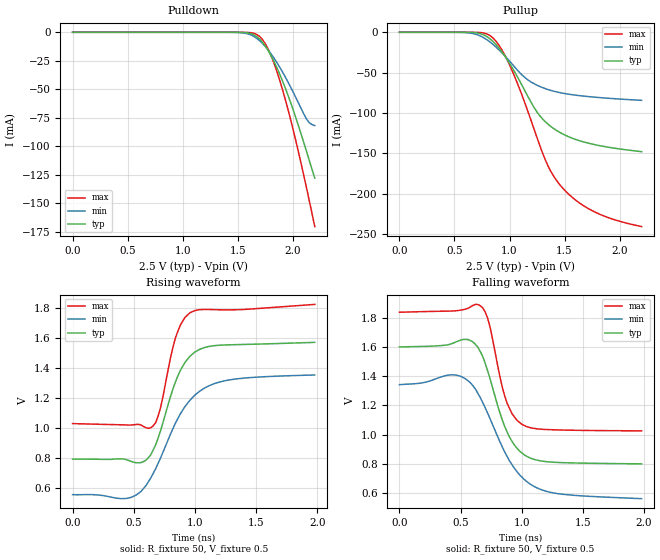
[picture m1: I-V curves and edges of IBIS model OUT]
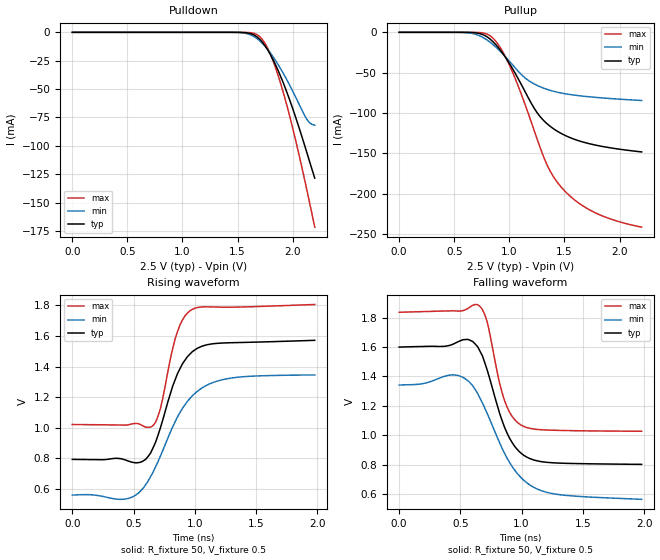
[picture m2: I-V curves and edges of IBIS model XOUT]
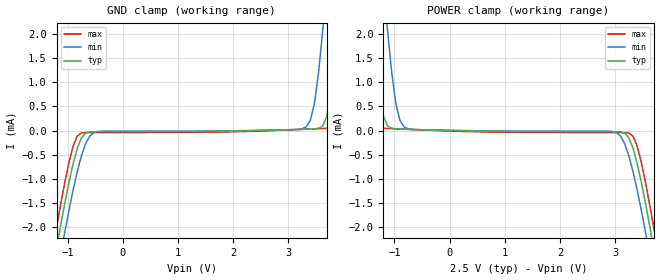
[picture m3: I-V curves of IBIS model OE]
|   IBIS File sg3225ean_25v.ibs
[IBIS Ver]   3.2
[File name]   sg3225ean_25v.ibs
[File Rev]   1.0
[Date]   May 1, 2013
[Source]
[Disclaimer]
Seiko Epson Corporation makes no warranty with respect to the information
contained herein.
[Copyright]
Copyright(C) 2013, Seiko Epson Corporation. All rights reserved.
|   Component SG3225EAN 2.5V
[Component]   sg3225ean_25v
[Manufacturer]   Seiko Epson Corporation
[Package]
R_pkg   0.048   NA   NA
L_pkg   0.48n   NA   NA
C_pkg   0.21p   NA   NA
[Pin] signal_name   model_name   R_pin   L_pin   C_pin
1   OE   OE
2   GND   GND
3   GND   GND
4   OUT   OUT   0.048   0.48n   0.21p
5   XOUT   XOUT   0.048   0.48n   0.21p
6   VCC   POWER
[Diff Pin] inv_pin vdiff   tdelay_typ
4   5   0   0
| Models and submodels in the file (3): OUT (Output_ECL), XOUT (Output_ECL), OE (Input)
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[Model]   OUT
Model_type Output_ECL
Enable Active-High
Polarity Non-Inverting
Vref=0.5
Vmeas=1.17
Rref=50
Cref=0
C_comp   0.121p   0.121p   0.121p
[Temperature Range] 25   105   -40
[Voltage Range]   2.5   2.25   2.75
[Pullup Reference]  2.5   2.25   2.75
[Pulldown Reference]2.5   2.25   2.75
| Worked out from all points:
|   falling waveform, R_fixture 50, V_fixture 0.5: 20-80 % time 196ps typ, 291ps min, 139ps max; typ from 1.6 V to 0.802 V
|   rising waveform, R_fixture 50, V_fixture 0.5: 20-80 % time 197ps typ, 299ps min, 137ps max; typ from 0.794 V to 1.57 V
[Pullup]
0V        611pA      1.028nA    671.3pA
625mV     -80.21uA   -627.6uA   -4.517uA
825mV     -8.344mA   -12.23mA   -4.283mA
900mV     -18.9mA    -21.18mA   -15.25mA
1V        -38.41mA   -35.67mA   -40.23mA
1.125V    -68.68mA   -54.32mA   -82.25mA
1.25V     -98.86mA   -65.59mA   -130.6mA
1.35V     -113.9mA   -70.95mA   -165.7mA
1.45V     -123.5mA   -74.53mA   -187.7mA
1.575V    -131.5mA   -77.43mA   -205.1mA
1.75V     -138.5mA   -80.07mA   -220.9mA
2.2V      -147.9mA   -84.31mA   -240.7mA
[Pulldown]
0V        611.1pA    1.029nA    671.4pA
1.5V      -32.97uA   -162.8uA   -2.785uA
1.625V    -1.356mA   -2.54mA    -453.5uA
1.7V      -6.054mA   -7.439mA   -3.728mA
1.75V     -12.01mA   -12.41mA   -9.925mA
1.8V      -20.03mA   -18.54mA   -19.8mA
1.85V     -29.76mA   -25.66mA   -32.69mA
1.9V      -40.95mA   -33.63mA   -47.96mA
2V        -66.91mA   -51.72mA   -83.97mA
2.125V    -104.4mA   -76.02mA   -136.4mA
2.15V     -112.3mA   -79.27mA   -147.5mA
2.2V      -127.8mA   -81.76mA   -170.3mA
[Falling Waveform]
R_fixture=50
V_fixture=0.5
V_fixture_min=0.25
V_fixture_max=0.75
0s        1.6V       1.342V     1.836V
460ps     1.633V     1.408V     1.846V
580ps     1.643V     1.355V     1.872V
680ps     1.537V     1.221V     1.867V
740ps     1.384V     1.111V     1.738V
840ps     1.103V     918.7mV    1.328V
880ps     1.019V     852.3mV    1.216V
1ns       876mV      711.6mV    1.072V
1.26ns    812.5mV    602.7mV    1.034V
1.98ns    801.5mV    563.8mV    1.027V
[Rising Waveform]
R_fixture=50
V_fixture=0.5
V_fixture_min=0.25
V_fixture_max=0.75
0s        794.5mV    558.3mV    1.03V
480ps     778.9mV    540.6mV    1.021V
580ps     778.1mV    599.2mV    1.011V
660ps     856.5mV    700.8mV    1.016V
720ps     985.1mV    803.3mV    1.138V
840ps     1.304V     1.032V     1.597V
880ps     1.381V     1.094V     1.683V
960ps     1.478V     1.186V     1.766V
1.24ns    1.552V     1.314V     1.786V
1.98ns    1.57V      1.353V     1.822V
[Ramp]
R_load=50
dV/dt_r   4.652E-1/1.974E-10   4.769E-1/2.992E-10   4.750E-1/1.371E-10
dV/dt_f   4.788E-1/1.963E-10   4.668E-1/2.907E-10   4.858E-1/1.390E-10
|[End   OUT
[Model]   XOUT
Model_type Output_ECL
Enable Active-High
Polarity Inverting
Vref=0.5
Vmeas=1.17
Rref=50
Cref=0
C_comp   0.121p   0.121p   0.121p
[Temperature Range] 25   105   -40
[Voltage Range]   2.5   2.25   2.75
[Pullup Reference]  2.5   2.25   2.75
[Pulldown Reference]2.5   2.25   2.75
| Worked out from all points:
|   falling waveform, R_fixture 50, V_fixture 0.5: 20-80 % time 194ps typ, 288ps min, 139ps max; typ from 1.6 V to 0.802 V
|   rising waveform, R_fixture 50, V_fixture 0.5: 20-80 % time 199ps typ, 293ps min, 134ps max; typ from 0.794 V to 1.57 V
[Pullup]
0V        610.9pA    1.028nA    671.1pA
625mV     -79.94uA   -626.2uA   -4.496uA
825mV     -8.35mA    -12.25mA   -4.281mA
900mV     -18.94mA   -21.22mA   -15.28mA
1V        -38.55mA   -35.75mA   -40.43mA
1.125V    -68.99mA   -54.45mA   -82.78mA
1.25V     -99.23mA   -65.7mA    -131.6mA
1.35V     -114.2mA   -71.07mA   -166.6mA
1.45V     -123.8mA   -74.65mA   -188.5mA
1.575V    -131.8mA   -77.55mA   -205.8mA
1.75V     -138.8mA   -80.2mA    -221.6mA
2.2V      -148.2mA   -84.46mA   -241.4mA
[Pulldown]
0V        611pA      1.028nA    671.2pA
1.5V      -32.54uA   -161.2uA   -2.736uA
1.625V    -1.345mA   -2.526mA   -448uA
1.7V      -6.028mA   -7.418mA   -3.701mA
1.75V     -11.99mA   -12.4mA    -9.894mA
1.8V      -20.02mA   -18.54mA   -19.8mA
1.85V     -29.8mA    -25.67mA   -32.76mA
1.9V      -41.04mA   -33.67mA   -48.14mA
2V        -67.16mA   -51.83mA   -84.44mA
2.125V    -104.9mA   -76.21mA   -137.3mA
2.15V     -112.8mA   -79.44mA   -148.6mA
2.2V      -128.4mA   -81.9mA    -171.6mA
[Falling Waveform]
R_fixture=50
V_fixture=0.5
V_fixture_min=0.25
V_fixture_max=0.75
0s        1.599V     1.341V     1.836V
480ps     1.635V     1.407V     1.844V
580ps     1.645V     1.355V     1.872V
660ps     1.571V     1.252V     1.876V
720ps     1.44V      1.146V     1.767V
820ps     1.15V      949.6mV    1.354V
860ps     1.055V     878.8mV    1.236V
1ns       874.7mV    707.2mV    1.067V
1.28ns    811.5mV    599mV      1.033V
1.98ns    801.9mV    564.1mV    1.027V
[Rising Waveform]
R_fixture=50
V_fixture=0.5
V_fixture_min=0.25
V_fixture_max=0.75
0s        794mV      561mV      1.021V
460ps     782.5mV    539.5mV    1.02V
580ps     784.2mV    606.9mV    1.011V
660ps     869.9mV    711.5mV    1.015V
720ps     1.001V     816.3mV    1.126V
800ps     1.22V      969.7mV    1.446V
860ps     1.355V     1.072V     1.63V
980ps     1.497V     1.209V     1.773V
1.26ns    1.555V     1.319V     1.787V
1.98ns    1.571V     1.345V     1.805V
[Ramp]
R_load=50
dV/dt_r   4.662E-1/1.991E-10   4.704E-1/2.935E-10   4.702E-1/1.337E-10
dV/dt_f   4.784E-1/1.943E-10   4.661E-1/2.881E-10   4.854E-1/1.390E-10
|[End   XOUT
[Model]   OE
Model_type Input
Vinh=1.75
Vinl=0.75
C_comp   3p   3p   3p
[Temperature Range] 25   105   -40
[Voltage Range]   2.5   2.25   2.75
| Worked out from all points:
|   GND clamp passes 1 mA (typ) near -0.96 V on its own axis
|   POWER clamp passes 1 mA (typ) near -1.29 V on its own axis
[GND Clamp]
-2.5V     -11.65mA   -12.17mA   -11.3mA
-1.2V     -2.439mA   -3.037mA   -2.004mA
-1.05V    -1.501mA   -2.093mA   -1.07mA
-750mV    -154.2uA   -526.6uA   -49.99uA
-450mV    -23.93uA   -19.15uA   -41.66uA
3.325V    27.94uA    75.78uA    27.31uA
3.475V    35.27uA    559.6uA    34.86uA
3.625V    94.02uA    2.074mA    42.53uA
3.7V      295.2uA    2.969mA    46.51uA
3.875V    2.014mA    5.059mA    78.18uA
4.175V    5.896mA    8.645mA    2.737mA
5V        16.61mA    18.53mA    14.18mA
[POWER Clamp]
-2.5V     16.61mA    18.53mA    14.18mA
-1.675V   5.896mA    8.645mA    2.737mA
-1.375V   2.014mA    5.059mA    78.18uA
-1.2V     295.2uA    2.969mA    46.51uA
-1.125V   94.02uA    2.074mA    42.53uA
-975mV    35.27uA    559.6uA    34.86uA
-825mV    27.94uA    75.78uA    27.31uA
2.95V     -23.93uA   -19.15uA   -41.66uA
3.25V     -154.2uA   -526.6uA   -49.99uA
3.55V     -1.501mA   -2.093mA   -1.07mA
3.7V      -2.439mA   -3.037mA   -2.004mA
5V        -11.65mA   -12.17mA   -11.3mA
